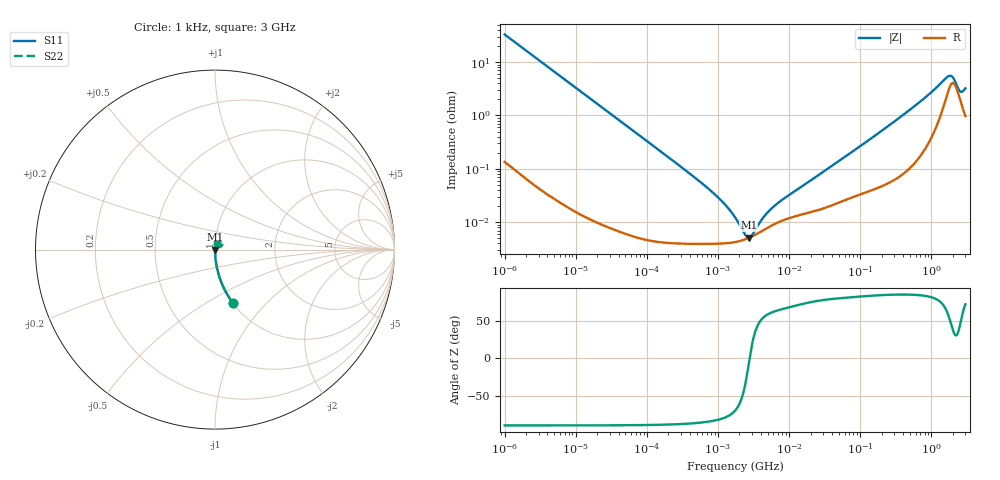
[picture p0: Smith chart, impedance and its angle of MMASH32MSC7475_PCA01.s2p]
! MMASH32MSC7475_PCA01  S-PARAMETER MODEL  ( Standard Model )
! Model Generated by TAIYO YUDEN Corporation (http://www.ty-top.com)
! Version 1.0
! TAIYO YUDEN Control No. 220601
! Copyright(c) 2016 TAIYO YUDEN CO.,LTD. All Rights Reserved.
! Product Description (link to TY-COMPAS)
! https://ds.yuden.co.jp/TYCOMPAS/or/detail?pn=MMASH32MSC7475KPCA01&u=M
! Products Name : Multilayer Ceramic Capacitors
! Characteristics :
!  Capacitance : 4.7 [uF] , Rated Voltage : 100 [V] , TCC : X7S
!  Case Size : 3.2 x 2.5 / 0.126 x 0.098 [mm/inch] , Thickness : 2.5 / 0.098 [mm/inch]
!  (Conditions: Temperature = 25 [degC] , DC Bias Voltage = 0 [V])
! External Node Assignments :
!  1  o---| |---o  2
! GND o---------o GND
! Frequency Range : 1kHz  -  3GHz  [ 401 STEP ]
# MHZ S RI R 50
! Freq[MHz].  S11 Real  S11 Imag  S21 Real  S21 Imag  S12 Real  S12 Imag  S22 Real  S22 Imag
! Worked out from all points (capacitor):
!   401 points, 1 kHz to 3 GHz, reference 50 ohm
!   read as one part in series: C = 4.84 uF near 1.077 kHz
!   lowest |Z| = 5.12 mohm at 2.709 MHz (marker M1)
!   series resonance near 2.776 MHz, so ESL is about 680 pH
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0.001  0.0984 -0.2958  0.9016 0.2958  0.9016 0.2958  0.0984 -0.2958
0.001685  0.0374 -0.1878  0.9626 0.1878  0.9626 0.1878  0.0374 -0.1878
0.00306  0.0119 -0.1063  0.9881 0.1063  0.9881 0.1063  0.0119 -0.1063
0.01216  0.000873 -0.0272  0.9991 0.0272  0.9991 0.0272  0.000873 -0.0272
0.147855  4.75e-05 -0.00224  1 0.00224  1 0.00224  4.75e-05 -0.00224
0.821683  3.95e-05 -0.000369  1 0.000369  1 0.000369  3.95e-05 -0.000369
1.285341  4.04e-05 -0.000203  1 0.000203  1 0.000203  4.04e-05 -0.000203
1.732051  4.25e-05 -0.000117  1 0.000117  1 0.000117  4.25e-05 -0.000117
2.010629  4.43e-05 -7.79e-05  1 7.79e-05  1 7.79e-05  4.43e-05 -7.79e-05
2.709407  5.08e-05 -5.6e-06  0.9999 5.6e-06  0.9999 5.6e-06  5.08e-05 -5.6e-06
3.651041  6.22e-05 6.24e-05  0.9999 -6.24e-05  0.9999 -6.24e-05  6.22e-05 6.24e-05
3.93371  6.59e-05 7.9e-05  0.9999 -7.9e-05  0.9999 -7.9e-05  6.59e-05 7.9e-05
5.30084  8.27e-05 0.000145  0.9999 -0.000145  0.9999 -0.000145  8.27e-05 0.000145
6.881678  9.86e-05 0.000204  0.9999 -0.000204  0.9999 -0.000204  9.86e-05 0.000204
21.06097  0.000157 0.000614  0.9998 -0.000614  0.9998 -0.000614  0.000157 0.000614
256.0921  0.000594 0.00655  0.9994 -0.00655  0.9994 -0.00655  0.000594 0.00655
727.4359  0.00223 0.0189  0.9978 -0.0189  0.9978 -0.0189  0.00223 0.0189
1714.862  0.0292 0.0434  0.9708 -0.0434  0.9708 -0.0434  0.0292 0.0434
1990.675  0.0401 0.0299  0.9599 -0.0299  0.9599 -0.0299  0.0401 0.0299
2489.759  0.0211 0.0186  0.9789 -0.0186  0.9789 -0.0186  0.0211 0.0186
2682.519  0.0156 0.0225  0.9844 -0.0225  0.9844 -0.0225  0.0156 0.0225
3000  0.0105 0.0301  0.9895 -0.0301  0.9895 -0.0301  0.0105 0.0301
